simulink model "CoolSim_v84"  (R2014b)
settings: Solver=ode1  StartTime=0.0  StopTime=trun  FixedStep=dtmax  MaxStep=dtmax  MinStep=1e-6  RelTol=1e-4
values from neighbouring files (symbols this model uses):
  aperp_cond = l_cond*gappl_cond - l_cond*densfin_cond*thfin_cond*lfin_cond    (= 0.00397716486616)    [CoolSim_v84_ec_init.m]    (also in CoolSim_v84_mc_init.m)
  apin_txv = 1e-3^2/4*pi    (= 7.85398163397e-07)    [CoolSim_v84_ec_init.m]    (also in CoolSim_v84_mc_init.m)
  area_cabinint = 8.0    (= 8)    [CoolSim_v84_ec_init.m]    (also in CoolSim_v84_mc_init.m)
  area_cabinshell = 4.0    (= 4)    [CoolSim_v84_ec_init.m]    (also in CoolSim_v84_mc_init.m)
  aseat_txv = dball_txv^2/4*pi    (= 7.06858347058e-06)    [CoolSim_v84_ec_init.m]    (also in CoolSim_v84_mc_init.m)
  atop_txv = 400e-6    (= 0.0004)    [CoolSim_v84_ec_init.m]    (also in CoolSim_v84_mc_init.m)
  c08 = -5.8002206e+003    (= -5800.2206)    [CoolSim_v84_ec_init.m]    (also in CoolSim_v84_mc_init.m)
  c09 = 1.3914993    [CoolSim_v84_ec_init.m]    (also in CoolSim_v84_mc_init.m)
  c10 = -4.8640239E-02    (= -0.048640239)    [CoolSim_v84_ec_init.m]    (also in CoolSim_v84_mc_init.m)
  c11 = 4.1764768E-05    (= 4.1764768e-05)    [CoolSim_v84_ec_init.m]    (also in CoolSim_v84_mc_init.m)
  c12 = -1.4452093E-08    (= -1.4452093e-08)    [CoolSim_v84_ec_init.m]    (also in CoolSim_v84_mc_init.m)
  c13 = 6.5459673    [CoolSim_v84_ec_init.m]    (also in CoolSim_v84_mc_init.m)
  c1_comprmech = 0.8728    [CoolSim_v84_ec_init.m]    (also in CoolSim_v84_mc_init.m = 0.9)
  c2_comprmech = 0.1777    [CoolSim_v84_ec_init.m]    (also in CoolSim_v84_mc_init.m = 0)
  cv_air = 719.    (= 719)    [CoolSim_v84_ec_init.m]    (also in CoolSim_v84_mc_init.m)
  deltat = 2e-4    (= 0.0002)    [CoolSim_v84_ec_init.m]    (also in CoolSim_v84_mc_init.m)
  dh_evaptocomp = 0.0    (= 0)    [CoolSim_v84_ec_init.m]    (also in CoolSim_v84_mc_init.m)
  displ_compr = 33e-6    (= 3.3e-05)    [CoolSim_v84_ec_init.m]    (also in CoolSim_v84_mc_init.m = 0.0002)
  dp_blower = [0,  40., 160., 360.]    [CoolSim_v84_ec_init.m]    (also in CoolSim_v84_mc_init.m)
  dp_evaptocomp = 0.0    (= 0)    [CoolSim_v84_ec_init.m]    (also in CoolSim_v84_mc_init.m)
  dpair_cond = 2300.    (= 2300)    [CoolSim_v84_ec_init.m]    (also in CoolSim_v84_mc_init.m)
  dt_evapout = 0.5    [CoolSim_v84_ec_init.m]    (also in CoolSim_v84_mc_init.m)
  dt_thermostat = 0.2    [CoolSim_v84_ec_init.m]    (also in CoolSim_v84_mc_init.m)
  eff_blower = 0.12    [CoolSim_v84_ec_init.m]    (also in CoolSim_v84_mc_init.m)
  eff_fan = 0.15    [CoolSim_v84_ec_init.m]    (also in CoolSim_v84_mc_init.m)
  einitvec_cond1 = 10.*ones(1,nseg_cond1)    [CoolSim_v84_ec_init.m]    (also in CoolSim_v84_mc_init.m)
  einitvec_cond2 = 10.*ones(1,nseg_cond2)    [CoolSim_v84_ec_init.m]    (also in CoolSim_v84_mc_init.m)
  einitvec_evap1 = 10.*ones(1,nseg_evap1)    [CoolSim_v84_ec_init.m]    (also in CoolSim_v84_mc_init.m)
  einitvec_evap2a = 10.*ones(1,nseg_evap2)    [CoolSim_v84_ec_init.m]    (also in CoolSim_v84_mc_init.m)
  einitvec_evap2b = 10.*ones(1,nseg_evap2)    [CoolSim_v84_ec_init.m]    (also in CoolSim_v84_mc_init.m)
  einitvec_evap3 = 10.*ones(1,nseg_evap3)    [CoolSim_v84_ec_init.m]    (also in CoolSim_v84_mc_init.m)
  einitvec_evap4 = 10.*ones(1,nseg_evap4)    [CoolSim_v84_ec_init.m]    (also in CoolSim_v84_mc_init.m)
  f1_blowcontr = -0.7    [CoolSim_v84_ec_init.m]    (also in CoolSim_v84_mc_init.m)
  f1_comprcontr = -0.02    [CoolSim_v84_ec_init.m]    (also in CoolSim_v84_mc_init.m)
  f2_blowcontr = 0.005    [CoolSim_v84_ec_init.m]    (also in CoolSim_v84_mc_init.m)
  f2_comprcontr = 1./6.    (= 0.166666666667)    [CoolSim_v84_ec_init.m]    (also in CoolSim_v84_mc_init.m)
  fp_txv = (psetbulb_txv - pset_txv)*atop_txv - 15e5*aseat_txv    [CoolSim_v84_ec_init.m]    (also in CoolSim_v84_mc_init.m)
  h_lookuphvsps = h1    [CoolSim_v84_ec_init.m]    (also in CoolSim_v84_mc_init.m)
  hmax_heater = 8000.    (= 8000)    [CoolSim_v84_ec_init.m]    (also in CoolSim_v84_mc_init.m)
  htin_enginecomp = 0.0    (= 0)    [CoolSim_v84_ec_init.m]    (also in CoolSim_v84_mc_init.m; point_ec01.m; point_mc01.m)
  htin_solarintvstime = [htin_solarint htin_solarint]    [CoolSim_v84_ec_init.m]    (also in CoolSim_v84_mc_init.m; point_ec01.m = [300. 300.]; point_mc01.m = [300. 300.])
  htin_solarshellvstime = [htin_solarshell htin_solarshell]    [CoolSim_v84_ec_init.m]    (also in CoolSim_v84_mc_init.m; point_ec01.m = [1000. 1000.]; point_mc01.m = [1000. 1000.])
  htrans_cabinint = 25.    (= 25)    [CoolSim_v84_ec_init.m]    (also in CoolSim_v84_mc_init.m)
  htrans_cabinshell = 15.    (= 15)    [CoolSim_v84_ec_init.m]    (also in CoolSim_v84_mc_init.m)
  ifmech = 0.0    (= 0)    [CoolSim_v84_ec_init.m]    (also in CoolSim_v84_mc_init.m = 1)
  iinitvec_cond1 = 0.0*ones(1,nseg_cond1+1)    [CoolSim_v84_ec_init.m]    (also in CoolSim_v84_mc_init.m)
  iinitvec_cond2 = 0.0*ones(1,nseg_cond2+1)    [CoolSim_v84_ec_init.m]    (also in CoolSim_v84_mc_init.m)
  iinitvec_evap1 = 0.0*ones(1,nseg_evap1+1)    [CoolSim_v84_ec_init.m]    (also in CoolSim_v84_mc_init.m)
  iinitvec_evap2a = 0.0*ones(1,nseg_evap2+1)    [CoolSim_v84_ec_init.m]    (also in CoolSim_v84_mc_init.m)
  iinitvec_evap2b = 0.0*ones(1,nseg_evap2+1)    [CoolSim_v84_ec_init.m]    (also in CoolSim_v84_mc_init.m)
  iinitvec_evap3 = 0.0*ones(1,nseg_evap3+1)    [CoolSim_v84_ec_init.m]    (also in CoolSim_v84_mc_init.m)
  iinitvec_evap4 = 0.0*ones(1,nseg_evap4+1)    [CoolSim_v84_ec_init.m]    (also in CoolSim_v84_mc_init.m)
  init_memrestart = 2250.    (= 2250)    [CoolSim_v84_ec_init.m]    (also in CoolSim_v84_mc_init.m; reinit.m = memrestart(n,2))
  init_picontr1 = 0.23    [CoolSim_v84_ec_init.m]    (also in CoolSim_v84_mc_init.m; reinit.m = picontr1(n,2))
  init_picontr2 = 0.32    [CoolSim_v84_ec_init.m]    (also in CoolSim_v84_mc_init.m; reinit.m = picontr2(n,2))
  iseff_rpm_pr = [0.650   0.728   0.717   0.655   0.569;     0.570   0.682   0.700   0.637   0.536;     0.460   0.590   0.650   0.600   0.493;     0.290   0.496   0.618   0.575   0.450]    [CoolSim_v84_ec_init.m]    (also in CoolSim_v84_mc_init.m = [0.8490    0.8490    0.7829    0.7409    0.7065    0.6802   )
  k_cabinleakin = 1e-4    (= 0.0001)    [CoolSim_v84_ec_init.m]    (also in CoolSim_v84_mc_init.m)
  k_cabinleakout = 4e-4    (= 0.0004)    [CoolSim_v84_ec_init.m]    (also in CoolSim_v84_mc_init.m)
  k_ram = 0.1    [CoolSim_v84_ec_init.m]    (also in CoolSim_v84_mc_init.m)
  l_cabinsurf = 2.0    (= 2)    [CoolSim_v84_ec_init.m]    (also in CoolSim_v84_mc_init.m)
  md_comprmax = rpm_max/60.*displ_compr*0.975*27.8    (= 0.10435425)    [CoolSim_v84_ec_init.m]    (also in CoolSim_v84_mc_init.m = 0.63245)
  minitvec_cond1 = 1e-4*ones(1,nseg_cond1)    [CoolSim_v84_ec_init.m]    (also in CoolSim_v84_mc_init.m)
  minitvec_cond2 = 1e-4*ones(1,nseg_cond2)    [CoolSim_v84_ec_init.m]    (also in CoolSim_v84_mc_init.m)
  minitvec_evap1 = 1e-4*ones(1,nseg_evap1)    [CoolSim_v84_ec_init.m]    (also in CoolSim_v84_mc_init.m)
  minitvec_evap2a = 1e-4*ones(1,nseg_evap2)    [CoolSim_v84_ec_init.m]    (also in CoolSim_v84_mc_init.m)
  minitvec_evap2b = 1e-4*ones(1,nseg_evap2)    [CoolSim_v84_ec_init.m]    (also in CoolSim_v84_mc_init.m)
  minitvec_evap3 = 1e-4*ones(1,nseg_evap3)    [CoolSim_v84_ec_init.m]    (also in CoolSim_v84_mc_init.m)
  minitvec_evap4 = 1e-4*ones(1,nseg_evap4)    [CoolSim_v84_ec_init.m]    (also in CoolSim_v84_mc_init.m)
  mrefr_outrate = 0.2    [CoolSim_v84_ec_init.m]    (also in CoolSim_v84_mc_init.m)
  mrefr_targ = 0.48    [CoolSim_v84_ec_init.m]    (also in CoolSim_v84_mc_init.m)
  nc1 = 35.    (= 35)    [CoolSim_v84_ec_init.m]    (also in CoolSim_v84_mc_init.m)
  nc2 = 9.0    (= 9)    [CoolSim_v84_ec_init.m]    (also in CoolSim_v84_mc_init.m)
  ne1 = 7.    (= 7)    [CoolSim_v84_ec_init.m]    (also in CoolSim_v84_mc_init.m)
  ne2a = 5.    (= 5)    [CoolSim_v84_ec_init.m]    (also in CoolSim_v84_mc_init.m)
  ne2b = 15.    (= 15)    [CoolSim_v84_ec_init.m]    (also in CoolSim_v84_mc_init.m)
  ne3 = 12.    (= 12)    [CoolSim_v84_ec_init.m]    (also in CoolSim_v84_mc_init.m)
  ne4 = 15.    (= 15)    [CoolSim_v84_ec_init.m]    (also in CoolSim_v84_mc_init.m)
  onoff_fanonoffvstime = [1  1]    [CoolSim_v84_ec_init.m]    (also in CoolSim_v84_mc_init.m; point_ec01.m; point_mc01.m)
  onoffinit_cabin = 1.0    (= 1)    [CoolSim_v84_ec_init.m]    (also in CoolSim_v84_mc_init.m; reinit.m = onoff_cabin(n,2))
  onoffinit_evap = 1.0    (= 1)    [CoolSim_v84_ec_init.m]    (also in CoolSim_v84_mc_init.m; reinit.m = onoff_evap(n,2))
  p_ambient = 1.013e5    (= 101300)    [CoolSim_v84_ec_init.m]    (also in CoolSim_v84_mc_init.m)
  p_ambvstime = [p_ambient p_ambient]    [CoolSim_v84_ec_init.m]    (also in CoolSim_v84_mc_init.m; point_ec01.m = [101300. 101300.]; point_mc01.m = [101300. 101300.])
  p_lookup_tsatvsp = psat*1e5    [CoolSim_v84_ec_init.m]    (also in CoolSim_v84_mc_init.m)
  r_h2o = 461.5043    [CoolSim_v84_ec_init.m]    (also in CoolSim_v84_mc_init.m)
  rair = 287.    (= 287)    [CoolSim_v84_ec_init.m]    (also in CoolSim_v84_mc_init.m)
  rate_txv = 35e3    (= 35000)    [CoolSim_v84_ec_init.m]    (also in CoolSim_v84_mc_init.m)
  ratio_compr = 1.37    [CoolSim_v84_ec_init.m]    (also in CoolSim_v84_mc_init.m)
  rh_ambvstime = [rh_ambient rh_ambient]    [CoolSim_v84_ec_init.m]    (also in CoolSim_v84_mc_init.m; point_ec01.m = [50. 50.]; point_mc01.m = [50. 50.])
  rpm_max = 7000.    (= 7000)    [CoolSim_v84_ec_init.m]    (also in CoolSim_v84_mc_init.m)
  rpm_minmaxrat = 1500./7000.    (= 0.214285714286)    [CoolSim_v84_ec_init.m]    (also in CoolSim_v84_mc_init.m)
  rpm_rpmvstime = [1600,  1600]    [CoolSim_v84_ec_init.m]    (also in CoolSim_v84_mc_init.m; point_mc01.m)
  rpm_switchoff = rpm_max*rpm_minmaxrat*1.01    (= 1515)    [CoolSim_v84_ec_init.m]    (also in CoolSim_v84_mc_init.m)
  s_txv = 0.8e-3    (= 0.0008)    [CoolSim_v84_ec_init.m]    (also in CoolSim_v84_mc_init.m)
  scfm_blower = [0, 100., 200., 300.]    [CoolSim_v84_ec_init.m]    (also in CoolSim_v84_mc_init.m)
  set_steadystate = 0.0    (= 0)    [CoolSim_v84_ec_init.m]    (also in CoolSim_v84_mc_init.m)
  setting_blend = 0.0    (= 0)    [CoolSim_v84_ec_init.m]    (also in CoolSim_v84_mc_init.m; point_mc01.m)
  setting_blower = 3.0    (= 3)    [CoolSim_v84_ec_init.m]    (also in CoolSim_v84_mc_init.m; point_mc01.m)
  setting_recirc = -1.0    (= -1)    [CoolSim_v84_ec_init.m]    (also in CoolSim_v84_mc_init.m; point_mc01.m = 0.95)
  shape_cabinsurf = 0.5    [CoolSim_v84_ec_init.m]    (also in CoolSim_v84_mc_init.m)
  smin_txv = 1e-6    (= 1e-06)    [CoolSim_v84_ec_init.m]    (also in CoolSim_v84_mc_init.m)
  t_ambvstime = [t_ambient t_ambient]    [CoolSim_v84_ec_init.m]    (also in CoolSim_v84_mc_init.m; point_ec01.m = [303.16 303.16]; point_mc01.m = [303.16 303.16])
  t_lookup_tsatvsp = t1    [CoolSim_v84_ec_init.m]    (also in CoolSim_v84_mc_init.m)
  tairevapout_limit = 274.    (= 274)    [CoolSim_v84_ec_init.m]    (also in CoolSim_v84_mc_init.m)
  tairin_cond = 303.16    [CoolSim_v84_ec_init.m]    (also in CoolSim_v84_mc_init.m; point_ec01.m; point_mc01.m)
  tbulbinit_txv = 273.0    (= 273)    [CoolSim_v84_ec_init.m]    (also in CoolSim_v84_mc_init.m; reinit.m = tbulb_txv(n,2))
  tchar_txv = 0.1    [CoolSim_v84_ec_init.m]    (also in CoolSim_v84_mc_init.m)
  tdel_cycling = 5.0    (= 5)    [CoolSim_v84_ec_init.m]    (also in CoolSim_v84_mc_init.m)
  tdelinit_cycling = 1.0    (= 1)    [CoolSim_v84_ec_init.m]    (also in CoolSim_v84_mc_init.m; reinit.m = tdel_cycling1(n,2))
  tevap_target = 273.16+3.0    (= 276.16)    [CoolSim_v84_ec_init.m]    (also in CoolSim_v84_mc_init.m)
  thmass_cabinint = 2e5    (= 200000)    [CoolSim_v84_ec_init.m]    (also in CoolSim_v84_mc_init.m)
  thmass_cabinshell = 1e5    (= 100000)    [CoolSim_v84_ec_init.m]    (also in CoolSim_v84_mc_init.m)
  time0 = 0.0    (= 0)    [CoolSim_v84_ec_init.m]    (also in CoolSim_v84_mc_init.m; reinit.m = time11(n,2))
  time_ambvstime = [0 1e5]    [CoolSim_v84_ec_init.m]    (also in CoolSim_v84_mc_init.m; point_ec01.m; point_mc01.m)
  time_fanonoffvstime = [0 1e5]    [CoolSim_v84_ec_init.m]    (also in CoolSim_v84_mc_init.m; point_ec01.m; point_mc01.m)
  time_rpmvstime = [0,    10000]    [CoolSim_v84_ec_init.m]    (also in CoolSim_v84_mc_init.m; point_mc01.m)
  time_solarintvstime = [0 1e5]    [CoolSim_v84_ec_init.m]    (also in CoolSim_v84_mc_init.m; point_ec01.m; point_mc01.m)
  time_solarshellvstime = [0 1e5]    [CoolSim_v84_ec_init.m]    (also in CoolSim_v84_mc_init.m; point_ec01.m; point_mc01.m)
  time_velvstime = [0 1e5]    [CoolSim_v84_ec_init.m]    (also in CoolSim_v84_mc_init.m; point_ec01.m; point_mc01.m)
  tinit_cabinint = 313.16    [CoolSim_v84_ec_init.m]    (also in CoolSim_v84_mc_init.m; point_ec01.m; point_mc01.m; reinit.m = t_cabinint(n,2))
  tinit_cabinshell = 308.16    [CoolSim_v84_ec_init.m]    (also in CoolSim_v84_mc_init.m; point_ec01.m; point_mc01.m; reinit.m = t_cabinshell(n,2))
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undefined symbols (not defined in the file or in its folder): nseg
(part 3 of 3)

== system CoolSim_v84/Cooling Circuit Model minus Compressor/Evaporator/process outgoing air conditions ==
  Divide : Product  Inputs=/*
  Divide1 : Product  Inputs=/*
  Mux : Mux  Inputs=5
  Mux1 : Mux  Inputs=3
  Mux2 : Mux  Inputs=3
  Terminator : Terminator
  add mass flow rates : Fcn  Expr=u(1)*ne1+u(5)*ne2a+u(9)*ne2b
  mass averaged relative humidity : Fcn  Expr=u(1)*u(3)*ne1+u(5)*u(7)*ne2a+u(9)*u(11)*ne2b
  mass averaged temperature : Fcn  Expr=u(1)*u(2)*ne1+u(5)*u(6)*ne2a+u(9)*u(10)*ne2b
  select T{,1..4} (5 alike) : Fcn  Expr=u(2)
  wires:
  select T4/1 -> Mux/3
  [airout_evap2b] -> select T4/1, Mux1/3
  select T2/1 -> Mux/4
  select T3/1 -> Mux/5
  [airout_evap4] -> select T3/1
  [airout_evap3] -> select T2/1
  [airout_evap2a] -> select T1/1, Mux1/2
  select T1/1 -> Mux/2
  select T/1 -> Mux/1
  [airout_evap1] -> Mux1/1, select T/1
  Mux/1 -> Terminator/1
  Mux1/1 -> add mass flow rates/1, mass averaged temperature/1, mass averaged relative humidity/1
  add mass flow rates/1 -> Divide/1, Divide1/1, Mux2/1
  Divide/1 -> Mux2/2
  mass averaged temperature/1 -> Divide/2
  mass averaged relative humidity/1 -> Divide1/2
  Divide1/1 -> Mux2/3
  Mux2/1 -> [evapout]

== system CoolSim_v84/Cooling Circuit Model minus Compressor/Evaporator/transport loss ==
  note: Only works for flow direction of evaporator to compressor
  qu : Inport
  pd : Inport  Port=2
  Demux : Demux  Outputs=2
  Demux1 : Demux
  Divide1 : Product  Inputs=**
  Divide2 : Product  Inputs=*/
  Mux : Mux  Inputs=2
  Mux1 : Mux
  Mux2 : Mux  Inputs=2
  Sum : Sum  Inputs=++|
  Sum1 : Sum  Inputs=|++
  adjust press drop : Constant  Value=dp_evaptocomp
  adjust press drop1 : Constant  Value=dh_evaptocomp
  ph_evapd : Scope
  qd : Outport
  pu : Outport  Port=2
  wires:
  Demux/1 -> Divide1/1, Mux/1, Divide2/2
  Demux1/2 -> Mux1/2
  Demux1/3 -> Mux1/3
  Demux1/4 -> Mux1/4
  qu/1 -> Demux/1
  Mux/1 -> qd/1
  pd/1 -> Demux1/1
  Mux1/1 -> pu/1
  Sum/1 -> Mux1/1, Mux2/1
  Demux1/1 -> Sum/2
  adjust press drop/1 -> Sum/1
  Demux/2 -> Sum1/1, Divide2/1
  adjust press drop1/1 -> Divide1/2
  Divide1/1 -> Sum1/2
  Sum1/1 -> Mux/2
  Mux2/1 -> ph_evapd/1
  Divide2/1 -> Mux2/2

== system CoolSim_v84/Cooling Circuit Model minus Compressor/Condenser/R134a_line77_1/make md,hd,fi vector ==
  vT : Inport
  Mux2 : Mux  Inputs=5
  Product : Product
  Product1 : Product
  Product2 : Product
  select air mass flow rate : Fcn  Expr=u(1)/nseg
  select mixture temperature : Fcn  Expr=u(2)
  select pmix_in : Fcn  Expr=u(3)
  select pmix_out : Fcn  Expr=u(4)
  select rel humidity : Fcn  Expr=u(5)
  vec : Constant  Value=ones(1,nseg)
  mdhdfvec : Outport
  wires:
  select pmix_out/1 -> Mux2/5
  select pmix_in/1 -> Mux2/4
  vT/1 -> select air mass flow rate/1, select pmix_out/1, select pmix_in/1, select rel humidity/1, select mixture temperature/1
  Mux2/1 -> mdhdfvec/1
  vec/1 -> Product/1, Product1/1, Product2/1
  Product1/1 -> Mux2/2
  Product/1 -> Mux2/1
  select air mass flow rate/1 -> Product/2
  select mixture temperature/1 -> Product1/2
  select rel humidity/1 -> Product2/2
  Product2/1 -> Mux2/3

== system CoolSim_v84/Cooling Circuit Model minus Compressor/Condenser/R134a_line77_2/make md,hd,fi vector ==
  vT : Inport
  Mux2 : Mux  Inputs=5
  Product : Product
  Product1 : Product
  Product2 : Product
  select air mass flow rate : Fcn  Expr=u(1)/nseg
  select mixture temperature : Fcn  Expr=u(2)
  select pmix_in : Fcn  Expr=u(3)
  select pmix_out : Fcn  Expr=u(4)
  select rel humidity : Fcn  Expr=u(5)
  vec : Constant  Value=ones(1,nseg)
  mdhdfvec : Outport
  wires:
  select pmix_out/1 -> Mux2/5
  select pmix_in/1 -> Mux2/4
  vT/1 -> select air mass flow rate/1, select pmix_out/1, select pmix_in/1, select rel humidity/1, select mixture temperature/1
  Mux2/1 -> mdhdfvec/1
  vec/1 -> Product/1, Product1/1, Product2/1
  Product1/1 -> Mux2/2
  Product/1 -> Mux2/1
  select air mass flow rate/1 -> Product/2
  select mixture temperature/1 -> Product1/2
  select rel humidity/1 -> Product2/2
  Product2/1 -> Mux2/3

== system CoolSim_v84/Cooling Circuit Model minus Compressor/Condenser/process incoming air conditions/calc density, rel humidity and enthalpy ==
  note: p/rho mix
  note: mix u spec
  press : Inport
  tempr : Inport  Port=2
  AH : Inport  Port=3
  Gain : Gain  Gain=cv_air
  Gain1 : Gain  Gain=100
  Mux : Mux  Inputs=3
  Mux1 : Mux  Inputs=2
  Product : Product
  Sum : Sum  Inputs=++|
  Sum1 : Sum  Inputs=+|+
  Sum2 : Sum  Inputs=-+|
  add : Sum
  air int energy : Product
  calc h2o vapor u spec : Fcn  Expr=(2501.3+1.82*(u(1)-273.16))*1000.
  calc psat_h2o : Fcn  Expr=exp(c08/u(1)+c09+c10*u(1)+c11*u(1)*u(1)+c12*u(1)*u(1)*u(1)+c13*log(u(1)))
  calc pure air density : Fcn  Expr=u(1)/rair/u(2)
  calc rel humidity : Fcn  Expr=u(3)*u(1)/(0.622+u(3))/u(2)
  div : Product  Inputs=/*
  div1 : Product  Inputs=/*
  h2o density : Product
  h2o int energy : Product
  one : Constant  Value=1.0
  p_h2o : Product
  dens : Outport
  RH : Outport  Port=2
  enth : Outport  Port=3
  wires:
  p_h2o/1 -> Sum2/1
  Sum2/1 -> Mux1/1
  Gain1/1 -> RH/1
  calc rel humidity/1 -> p_h2o/2, Gain1/1
  add/1 -> enth/1
  div1/1 -> add/2
  div/1 -> add/1
  Sum1/1 -> div/2
  calc h2o vapor u spec/1 -> h2o int energy/2
  h2o density/1 -> h2o int energy/1
  h2o int energy/1 -> Sum1/2
  Gain/1 -> air int energy/2
  air int energy/1 -> Sum1/1
  Product/1 -> div1/1, div/1, dens/1
  one/1 -> Sum/2
  Sum/1 -> Product/1
  calc pure air density/1 -> Product/2, h2o density/2, air int energy/1
  Mux1/1 -> calc pure air density/1
  calc psat_h2o/1 -> p_h2o/1, Mux/2
  Mux/1 -> calc rel humidity/1
  press/1 -> Sum2/2, div1/2, Mux/1
  AH/1 -> h2o density/1, Sum/1, Mux/3
  tempr/1 -> calc h2o vapor u spec/1, Gain/1, Mux1/2, calc psat_h2o/1

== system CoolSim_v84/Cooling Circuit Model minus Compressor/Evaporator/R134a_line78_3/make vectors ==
  mdtppf : Inport
  Mux2 : Mux  Inputs=5
  Product : Product
  Product1 : Product
  Product2 : Product
  select air mass flow rate : Fcn  Expr=u(1)/nseg
  select mixture temperature : Fcn  Expr=u(2)
  select pmix_in : Fcn  Expr=u(3)
  select pmix_out : Fcn  Expr=u(4)
  select rel humidity : Fcn  Expr=u(5)
  vec : Constant  Value=ones(1,nseg)
  vector : Outport
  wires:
  select pmix_out/1 -> Mux2/5
  select pmix_in/1 -> Mux2/4
  mdtppf/1 -> select air mass flow rate/1, select pmix_out/1, select pmix_in/1, select rel humidity/1, select mixture temperature/1
  Mux2/1 -> vector/1
  vec/1 -> Product/1, Product1/1, Product2/1
  Product1/1 -> Mux2/2
  Product/1 -> Mux2/1
  select air mass flow rate/1 -> Product/2
  select mixture temperature/1 -> Product1/2
  select rel humidity/1 -> Product2/2
  Product2/1 -> Mux2/3

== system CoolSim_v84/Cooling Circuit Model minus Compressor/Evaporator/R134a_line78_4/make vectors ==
  mdtppf : Inport
  Mux2 : Mux  Inputs=5
  Product : Product
  Product1 : Product
  Product2 : Product
  select air mass flow rate : Fcn  Expr=u(1)/nseg
  select mixture temperature : Fcn  Expr=u(2)
  select pmix_in : Fcn  Expr=u(3)
  select pmix_out : Fcn  Expr=u(4)
  select rel humidity : Fcn  Expr=u(5)
  vec : Constant  Value=ones(1,nseg)
  vector : Outport
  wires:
  select pmix_out/1 -> Mux2/5
  select pmix_in/1 -> Mux2/4
  mdtppf/1 -> select air mass flow rate/1, select pmix_out/1, select pmix_in/1, select rel humidity/1, select mixture temperature/1
  Mux2/1 -> vector/1
  vec/1 -> Product/1, Product1/1, Product2/1
  Product1/1 -> Mux2/2
  Product/1 -> Mux2/1
  select air mass flow rate/1 -> Product/2
  select mixture temperature/1 -> Product1/2
  select rel humidity/1 -> Product2/2
  Product2/1 -> Mux2/3
